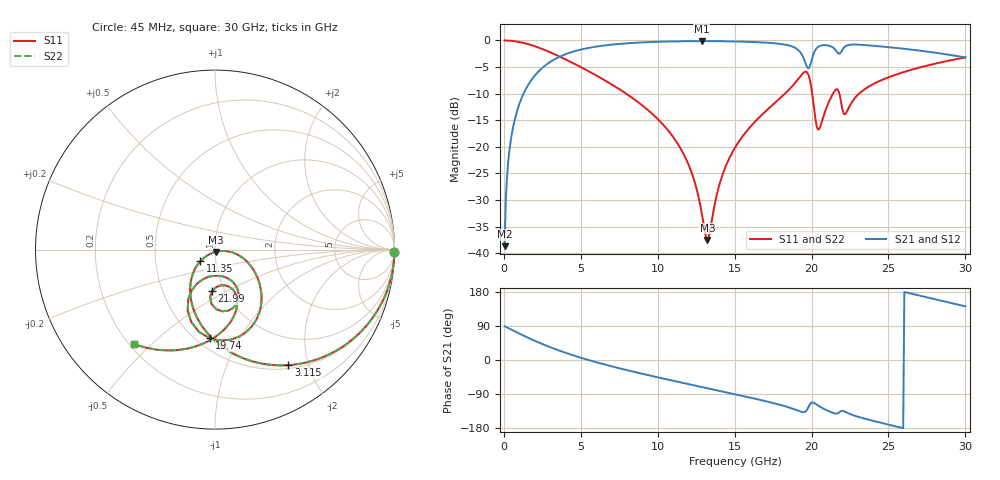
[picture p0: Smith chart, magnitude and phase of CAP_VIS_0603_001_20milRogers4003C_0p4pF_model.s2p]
! S-parameter model data by Modelithics Inc.  support@modelithics.com  813-866-6335  Tampa FL USA
! S-Parameter data specifications:
! Substrate: 20-mil Rogers 4003C, substrate thickness, H=0.508mm, Dielectric constant, Er=3.75
! PCB Mounting Pad Footprint: Pad width, PadW=0.90mm , Pad length, PadL=1.00mm , Pad gap, PadG (edge-to-edge)=1.00mm , Reference planes=3.0mm apart
! Created Wed Nov 18 13:16:16 2015
# hz S ma R 50
! 2 Port Network Data from SP1.SP block
! freq  magS11  angS11  magS21  angS21  magS12  angS12  magS22  angS22
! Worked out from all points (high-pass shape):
!   401 points, 45 MHz to 30 GHz, reference 50 ohm
!   highest |S21| = -0.13 dB at 12.85 GHz (marker M1); lowest = -38.7 dB at 45 MHz (marker M2)
!   |S21| within 3 dB of the highest: 3.568 GHz to 19.45 GHz (15.88 GHz wide, 138 % of centre); 20.06 GHz to 29.85 GHz (9.794 GHz wide, 39.2 % of centre)
!   lowest |S11| = -37.5 dB at 13.23 GHz (marker M3), VSWR 1.03, Z = 50.3 - j1.3 ohm
!   |S11| at or under -10 dB: 7.948 GHz to 18.27 GHz (10.32 GHz wide, 78.7 % of centre); 20.04 GHz to 21.39 GHz (1.349 GHz wide, 6.51 % of centre); 21.8 GHz to 23.09 GHz (1.282 GHz wide, 5.71 % of centre)
!   |S22| runs from -37.5 to 0.0 dB; largest |S21 - S12| = 0
!   S11 on the Smith chart (normalised r, x): 45 MHz: open; 3.115 GHz: 0.55, -1.68; 11.35 GHz: 0.84, -0.11; 19.74 GHz: 0.58, -0.76; 21.99 GHz: 0.87, -0.43; 30 GHz: 0.22, -0.44
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4.5e7  0.9999 -0.9  0.01167 89.1  0.01167 89.1  0.9999 -0.9
3.4455e8  0.996 -7.1  0.08907 82.9  0.08907 82.9  0.996 -7.1
8.687625e8  0.9752 -17.6  0.2205 72.3  0.2205 72.3  0.9752 -17.6
3.115388e9  0.7623 -57.6  0.6432 32.1  0.6432 32.1  0.7623 -57.6
5.062462e9  0.5556 -84.1  0.8251 5.2  0.8251 5.2  0.5556 -84.1
7.309088e9  0.363 -108.6  0.923 -19.8  0.923 -19.8  0.363 -108.6
1.007992e10  0.1777 -133.1  0.9727 -46.5  0.9727 -46.5  0.1777 -133.1
1.135301e10  0.1039 -141.5  0.982 -57.9  0.982 -57.9  0.1039 -141.5
1.225166e10  0.05469 -142.8  0.9851 -65.9  0.9851 -65.9  0.05469 -142.8
1.285076e10  0.02434 -128.9  0.9856 -71.2  0.9856 -71.2  0.02434 -128.9
1.32252e10  0.01336 -75.9  0.9854 -74.5  0.9854 -74.5  0.01336 -75.9
1.412385e10  0.05021 -8.9  0.9832 -82.4  0.9832 -82.4  0.05021 -8.9
1.50225e10  0.0983 -9.4  0.9784 -90.3  0.9784 -90.3  0.0983 -9.4
1.891665e10  0.3973 -49.6  0.8547 -130.5  0.8547 -130.5  0.3973 -49.6
1.974041e10  0.4948 -93.5  0.5528 -128.9  0.5528 -128.9  0.4948 -93.5
2.003996e10  0.3162 -118.2  0.6831 -112.0  0.6831 -112.0  0.3162 -118.2
2.048929e10  0.1466 -82.2  0.8809 -122.0  0.8809 -122.0  0.1466 -82.2
2.153771e10  0.3409 -73.1  0.8201 -141.4  0.8201 -141.4  0.3409 -73.1
2.198704e10  0.2318 -93.9  0.8096 -134.2  0.8096 -134.2  0.2318 -93.9
2.296058e10  0.3036 -66.1  0.9139 -149.0  0.9139 -149.0  0.3036 -66.1
2.505742e10  0.4537 -84.4  0.8635 -171.2  0.8635 -171.2  0.4537 -84.4
3e10  0.6925 -130.6  0.6918 141.5  0.6918 141.5  0.6925 -130.6
